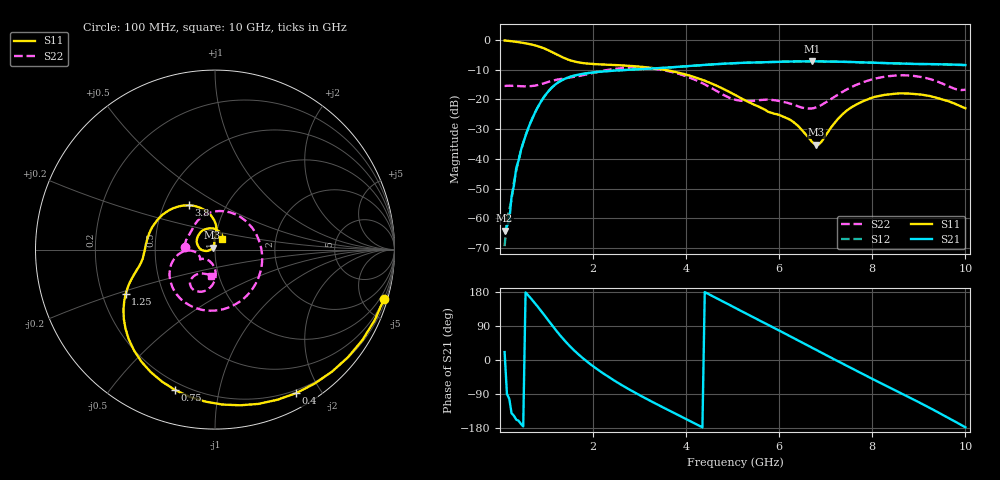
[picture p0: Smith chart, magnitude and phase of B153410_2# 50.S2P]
!  2-Port S-parameters saved by WinCal
! VAR MeasName=S-Parameters (CALIBRATED_DATA) read from VNA (N5245A)
! VAR MeasDate=2016-12-23 10:02:00
! VAR NAME=B153410_2# 50
! VAR FILENAME=B153410_2# 50.S2P
! VAR DATE=2016-12-23 10:02:00
! VAR PHYS_PORTS=1,2
# Hz S DB R 50
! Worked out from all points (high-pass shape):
!   199 points, 100 MHz to 10 GHz, reference 50 ohm
!   highest |S21| = -7.17 dB at 6.7 GHz (marker M1); lowest = -64.1 dB at 100 MHz (marker M2)
!   |S21| within 3 dB of the highest: 2.593 GHz to end of sweep
!   lowest |S11| = -35.2 dB at 6.8 GHz (marker M3), VSWR 1.04, Z = 48.7 + j1.06 ohm
!   |S11| at or under -10 dB: 3.522 GHz to end of sweep
!   |S22| runs from -23.0 to -9.3 dB; largest |S21 - S12| = 0.0025
!   S11 on the Smith chart (normalised r, x): 100 MHz: 0.47, -6.98; 400 MHz: 0.17, -1.70; 750 MHz: 0.16, -0.74; 1.25 GHz: 0.30, -0.21; 3.8 GHz: 0.67, +0.36; 10 GHz: 1.08, +0.13
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1e8  -0.16 -16.2  -64.12 20.9  -69.33 66.4  -15.46 175.4
1.5e8  -0.24 -24.0  -62.68 -89.7  -60.37 -55.7  -15.41 172.5
2e8  -0.32 -31.5  -60.76 -102.5  -57.06 -126.6  -15.37 169.4
2.5e8  -0.42 -38.9  -52.57 -140.6  -53.70 -129.6  -15.42 166.3
4e8  -0.74 -60.5  -40.49 -160.2  -40.59 -157.6  -15.48 157.5
7.5e8  -1.80 -106.0  -24.52 149.9  -24.54 150.2  -15.38 137.4
1e9  -3.17 -133.7  -18.05 110.8  -18.00 110.9  -14.28 115.9
1.25e9  -5.11 -153.6  -14.28 71.3  -14.24 71.3  -13.27 82.8
1.75e9  -7.69 -171.2  -11.48 8.0  -11.46 8.0  -11.95 8.5
2.55e9  -8.48 165.4  -10.21 -61.3  -10.21 -61.4  -9.57 -78.2
3.4e9  -9.69 135.4  -9.49 -118.5  -9.49 -118.6  -9.88 -135.9
3.8e9  -10.86 120.6  -9.05 -143.5  -9.06 -143.5  -11.20 -156.1
4.45e9  -14.00 98.5  -8.32 175.9  -8.35 175.9  -15.35 -177.1
5.05e9  -18.48 86.2  -7.79 137.8  -7.81 137.9  -20.08 -166.5
5.9e9  -24.82 93.3  -7.39 84.1  -7.37 84.1  -20.25 -146.0
6.3e9  -27.53 95.4  -7.24 58.4  -7.25 58.5  -21.69 -140.8
6.7e9  -34.17 117.7  -7.17 32.8  -7.19 32.8  -23.02 -116.7
6.8e9  -35.25 140.8  -7.18 26.3  -7.20 26.4  -22.62 -108.7
7.5e9  -23.18 -176.7  -7.37 -18.4  -7.39 -18.5  -16.23 -89.0
8.35e9  -18.30 141.1  -7.84 -71.4  -7.85 -71.5  -12.17 -107.8
9.15e9  -18.58 93.8  -8.08 -121.0  -8.13 -121.0  -12.79 -127.5
1e10  -22.95 54.6  -8.43 -177.7  -8.48 -177.5  -16.70 -99.1
